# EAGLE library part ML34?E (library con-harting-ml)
HARTING
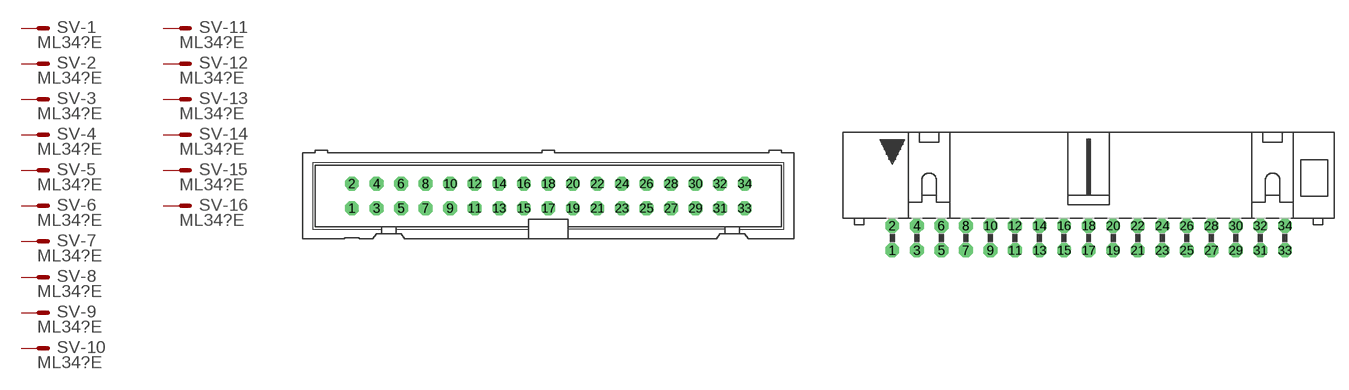
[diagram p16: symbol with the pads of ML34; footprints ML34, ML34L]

Designator prefix SV; gates -1=M -2=M -3=M -4=M -5=M -6=M -7=M -8=M -9=M -10=M -11=M -12=M -13=M -14=M -15=M -16=M -17=M -18=M -19=M -20=M -21=M -22=M -23=M -24=M -25=M -26=M -27=M -28=M -29=M -30=M -31=M -32=M -33=M -34=M

## ML34E (OC_FARNELL: unknown; OC_NEWARK: unknown)  [ML34]
1  -1:S  pas
2  -2:S  pas
3  -3:S  pas
4  -4:S  pas
5  -5:S  pas
6  -6:S  pas
7  -7:S  pas
8  -8:S  pas
9  -9:S  pas
10  -10:S  pas
11  -11:S  pas
12  -12:S  pas
13  -13:S  pas
14  -14:S  pas
15  -15:S  pas
16  -16:S  pas
17  -17:S  pas
18  -18:S  pas
19  -19:S  pas
20  -20:S  pas
21  -21:S  pas
22  -22:S  pas
23  -23:S  pas
24  -24:S  pas
25  -25:S  pas
26  -26:S  pas
27  -27:S  pas
28  -28:S  pas
29  -29:S  pas
30  -30:S  pas
31  -31:S  pas
32  -32:S  pas
33  -33:S  pas
34  -34:S  pas

## ML34LE (OC_FARNELL: unknown; OC_NEWARK: unknown)  [ML34L]
Pads as for ML34

## ML343ME (OC_FARNELL: unknown; OC_NEWARK: unknown)  [3M_34]
Pads as for ML34

## ML343MLE (OC_FARNELL: unknown; OC_NEWARK: unknown)  [3M_34L]
Pads as for ML34

## Footprint ML34 (pad centres in mm)
HARTING
drill 0.914 octagon: 1 -20.32,-1.27; 2 -20.32,1.27; 3 -17.78,-1.27; 4 -17.78,1.27; 5 -15.24,-1.27; 6 -15.24,1.27; 7 -12.7,-1.27; 8 -12.7,1.27; 9 -10.16,-1.27; 10 -10.16,1.27; 11 -7.62,-1.27; 12 -7.62,1.27; 13 -5.08,-1.27; 14 -5.08,1.27; 15 -2.54,-1.27; 16 -2.54,1.27; 17 0,-1.27; 18 0,1.27; 19 2.54,-1.27; 20 2.54,1.27; 21 5.08,-1.27; 22 5.08,1.27; 23 7.62,-1.27; 24 7.62,1.27; 25 10.16,-1.27; 26 10.16,1.27; 27 12.7,-1.27; 28 12.7,1.27; 29 15.24,-1.27; 30 15.24,1.27; 31 17.78,-1.27; 32 17.78,1.27; 33 20.32,-1.27; 34 20.32,1.27

## Footprint ML34L (pad centres in mm)
HARTING
drill 0.914 octagon: 1 -20.32,-1.27; 2 -20.32,1.27; 3 -17.78,-1.27; 4 -17.78,1.27; 5 -15.24,-1.27; 6 -15.24,1.27; 7 -12.7,-1.27; 8 -12.7,1.27; 9 -10.16,-1.27; 10 -10.16,1.27; 11 -7.62,-1.27; 12 -7.62,1.27; 13 -5.08,-1.27; 14 -5.08,1.27; 15 -2.54,-1.27; 16 -2.54,1.27; 17 0,-1.27; 18 0,1.27; 19 2.54,-1.27; 20 2.54,1.27; 21 5.08,-1.27; 22 5.08,1.27; 23 7.62,-1.27; 24 7.62,1.27; 25 10.16,-1.27; 26 10.16,1.27; 27 12.7,-1.27; 28 12.7,1.27; 29 15.24,-1.27; 30 15.24,1.27; 31 17.78,-1.27; 32 17.78,1.27; 33 20.32,-1.27; 34 20.32,1.27

## Footprint 3M_34 (pad centres in mm)
3M
drill 0.813 square: 1 -20.32,-1.27; 2 -20.32,1.27; 3 -17.78,-1.27; 4 -17.78,1.27; 5 -15.24,-1.27; 6 -15.24,1.27; 7 -12.7,-1.27; 8 -12.7,1.27; 9 -10.16,-1.27; 10 -10.16,1.27; 11 -7.62,-1.27; 12 -7.62,1.27; 13 -5.08,-1.27; 14 -5.08,1.27; 15 -2.54,-1.27; 16 -2.54,1.27; 17 0,-1.27; 18 0,1.27; 19 2.54,-1.27; 20 2.54,1.27; 21 5.08,-1.27; 22 5.08,1.27; 23 7.62,-1.27; 24 7.62,1.27; 25 10.16,-1.27; 26 10.16,1.27; 27 12.7,-1.27; 28 12.7,1.27; 29 15.24,-1.27; 30 15.24,1.27; 31 17.78,-1.27; 32 17.78,1.27; 33 20.32,-1.27; 34 20.32,1.27

## Footprint 3M_34L (pad centres in mm)
3M
drill 0.813 square: 1 -20.32,-5.08; 2 -20.32,-2.54; 3 -17.78,-5.08; 4 -17.78,-2.54; 5 -15.24,-5.08; 6 -15.24,-2.54; 7 -12.7,-5.08; 8 -12.7,-2.54; 9 -10.16,-5.08; 10 -10.16,-2.54; 11 -7.62,-5.08; 12 -7.62,-2.54; 13 -5.08,-5.08; 14 -5.08,-2.54; 15 -2.54,-5.08; 16 -2.54,-2.54; 17 0,-5.08; 18 0,-2.54; 19 2.54,-5.08; 20 2.54,-2.54; 21 5.08,-5.08; 22 5.08,-2.54; 23 7.62,-5.08; 24 7.62,-2.54; 25 10.16,-5.08; 26 10.16,-2.54; 27 12.7,-5.08; 28 12.7,-2.54; 29 15.24,-5.08; 30 15.24,-2.54; 31 17.78,-5.08; 32 17.78,-2.54; 33 20.32,-5.08; 34 20.32,-2.54
hole 2.54 at -26.238,-3.277
hole 2.54 at 26.238,-3.277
